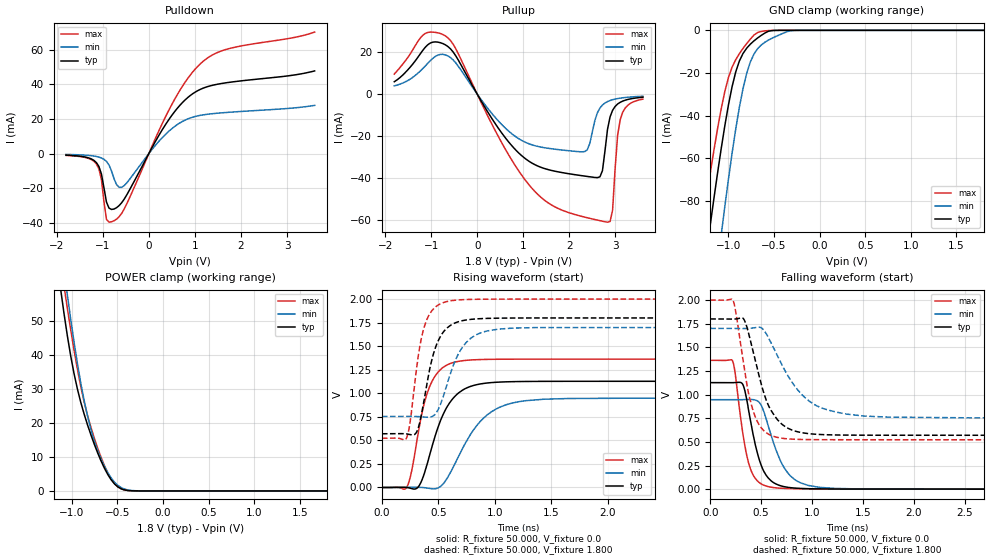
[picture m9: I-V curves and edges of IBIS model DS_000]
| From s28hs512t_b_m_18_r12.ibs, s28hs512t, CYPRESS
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|   Model DS_000
[Model] DS_000
Model_type 3-state
Polarity   Non-Inverting
Enable   Active-High
Vmeas =  0.900V
Cref =  15.000pF
C_comp   5.334pF   5.23pF   5.767pF
[Temperature Range]   25.000   0.125k   -40.000
[Voltage Range]   1.800V   1.700V   2.000V
[Pullup Reference]   1.800V   1.700V   2.000V
[Pulldown Reference]   0.0V   0.0V   0.0V
[POWER Clamp Reference]   1.800V   1.700V   2.000V
[GND Clamp Reference]   0.0V   0.0V   0.0V
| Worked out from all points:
|   slope of the pulldown table from 0 to 0.27 V, typ, clamps not added: 21 ohm
|   slope of the pullup table from 0 to 0.27 V, typ, clamps not added: 27.1 ohm
|   GND clamp passes 1 mA (typ) near -0.59 V on its own axis
|   POWER clamp passes 1 mA (typ) near -0.48 V on its own axis
|   rising waveform, R_fixture 50.000, V_fixture 0.0: 20-80 % time 207ps typ, 300ps min, 151ps max; typ from 0 V to 1.13 V
|   rising waveform, R_fixture 50.000, V_fixture 1.800: 20-80 % time 141ps typ, 191ps min, 112ps max; typ from 0.57 V to 1.8 V
|   falling waveform, R_fixture 50.000, V_fixture 0.0: 20-80 % time 144ps typ, 205ps min, 117ps max; typ from 1.13 V to 0 V
|   falling waveform, R_fixture 50.000, V_fixture 1.800: 20-80 % time 209ps typ, 344ps min, 149ps max; typ from 1.8 V to 0.57 V
[Pulldown]
|Voltage   I(typ)   I(min)   I(max)
-1.8V     -919.4uA   -496.1uA   -1.054mA
-1.14V    -5.184mA   -1.692mA   -5.957mA
-1.03V    -11.81mA   -2.55mA    -15.02mA
-920mV    -28.09mA   -4.545mA   -38.04mA
-755mV    -32.07mA   -14.63mA   -38.83mA
-645mV    -30.07mA   -19.53mA   -36.53mA
-535mV    -26.34mA   -18.54mA   -32.06mA
455mV     20.46mA    13.41mA    26.17mA
785mV     30.97mA    19.33mA    41.2mA
1.115V    37.1mA     22.09mA    51.84mA
1.72V     41.1mA     23.84mA    60.55mA
3.6V      47.81mA    27.87mA    70.26mA
[Pullup]
|Voltage   I(typ)   I(min)   I(max)
-1.8V     5.887mA    3.895mA    9.515mA
-1.13V    22.22mA    13.31mA    28.84mA
-690mV    23.43mA    18.67mA    27.68mA
575mV     -19.78mA   -15.44mA   -24.84mA
1.235V    -33.42mA   -24.47mA   -45.96mA
2.335V    -39.05mA   -27.38mA   -58.59mA
2.665V    -39.41mA   -6.666mA   -60.27mA
2.83V     -16.78mA   -3.58mA    -61.01mA
2.94V     -7.734mA   -2.688mA   -55.31mA
3.05V     -4.724mA   -2.141mA   -19.48mA
3.105V    -3.923mA   -1.94mA    -12.23mA
3.6V      -1.506mA   -1.042mA   -2.402mA
[GND_clamp]
|Voltage   I(typ)   I(min)   I(max)
-1.8V     -294mA     -373mA     -247.3mA
-1.28V    -116.8mA   -168.5mA   -89.46mA
-1.2V     -91.34mA   -138.7mA   -67.04mA
-1.08V    -55.6mA    -96.11mA   -36.91mA
-1.04V    -44.83mA   -82.66mA   -28.74mA
-1V       -34.98mA   -69.76mA   -22.14mA
-920mV    -19.48mA   -46.23mA   -13.73mA
-800mV    -8.377mA   -20.18mA   -6.205mA
-680mV    -3.579mA   -8.59mA    -1.029mA
-560mV    -408.3uA   -4.544mA   -113.8uA
-280mV    -162.8nA   -73.51uA   -82.13nA
1.8V      272.8pA    325nA      188.3pA
[POWER_clamp]
|Voltage   I(typ)   I(min)   I(max)
-1.8V     236.7mA    239.1mA    251.1mA
-1.123V   59.68mA    73.25mA    67.66mA
-1.086V   52.46mA    65.42mA    60.6mA
-1.049V   45.83mA    57.89mA    53.9mA
-938mV    30.03mA    37.57mA    35.87mA
-864mV    22.62mA    26.6mA     26.18mA
-790mV    16.52mA    18.14mA    18.76mA
-716mV    11.21mA    11.92mA    12.63mA
-642mV    6.708mA    7.258mA    7.47mA
-494mV    1.178mA    1.619mA    1.205mA
-272mV    6.291uA    28.11uA    4.439uA
1.8V      0A         0A         0A
[Ramp]
| variable   typ   min   max
dV/dt_r   0.676/0.206n   0.568/0.300n   0.817/0.151n
dV/dt_f   0.738/0.209n   0.568/0.344n   0.887/0.149n
R_load = 50.000
[Rising Waveform]
R_fixture= 50.000
V_fixture= 0.0
V_fixture_min= 0.0
V_fixture_max= 0.0
|time   V(typ)   V(min)   V(max)
0s        3.147uV    4.171uV    4.879uV
221ps     -252.8uV   900.2uV    2.694mV
323ps     6.313mV    1.633mV    585.3mV
386ps     189.5mV    -3.823mV   940.1mV
451ps     463.1mV    -14.34mV   1.142V
558ps     813.4mV    61.15mV    1.288V
680ps     1.004V     331.9mV    1.339V
931ps     1.109V     768.5mV    1.36V
1.271ns   1.125V     920.9mV    1.362V
6ns       1.127V     946.7mV    1.362V
[Rising Waveform]
R_fixture= 50.000
V_fixture= 1.800
V_fixture_min= 1.700
V_fixture_max= 2.000
|time   V(typ)   V(min)   V(max)
0s        570mV      753.8mV    522.4mV
218ps     568.7mV    754.6mV    524.5mV
251ps     561.4mV    754.5mV    700.4mV
308ps     588.6mV    753.2mV    1.272V
409ps     1.167V     745.3mV    1.811V
487ps     1.525V     802.4mV    1.928V
582ps     1.698V     1.115V     1.975V
738ps     1.776V     1.527V     1.995V
1.032ns   1.797V     1.681V     1.999V
6ns       1.8V       1.7V       2V
[Falling Waveform]
R_fixture= 50.000
V_fixture= 0.0
V_fixture_min= 0.0
V_fixture_max= 0.0
|time   V(typ)   V(min)   V(max)
0s        1.127V     946.6mV    1.362V
219ps     1.126V     946.2mV    1.358V
247ps     1.127V     946.2mV    1.214V
319ps     1.11V      946.7mV    600.3mV
412ps     630.5mV    948.1mV    169.9mV
498ps     261mV      892.8mV    58.08mV
593ps     92.93mV    589.6mV    21.56mV
786ps     16.17mV    142.3mV    6.386mV
1.072ns   2.812mV    19.53mV    2.756mV
6ns       2.282uV    16.16uV    -1.321uV
[Falling Waveform]
R_fixture= 50.000
V_fixture= 1.800
V_fixture_min= 1.700
V_fixture_max= 2.000
|time   V(typ)   V(min)   V(max)
0s        1.8V       1.7V       2V
224ps     1.799V     1.7V       1.998V
328ps     1.801V     1.699V     1.327V
380ps     1.636V     1.7V       996.1mV
452ps     1.323V     1.71V      739.5mV
551ps     939.2mV    1.643V     596.6mV
661ps     733.9mV    1.409V     546.9mV
967ps     587.2mV    935.3mV    524.2mV
1.343ns   571.7mV    792.9mV    522.6mV
6ns       570mV      753.8mV    522.4mV
